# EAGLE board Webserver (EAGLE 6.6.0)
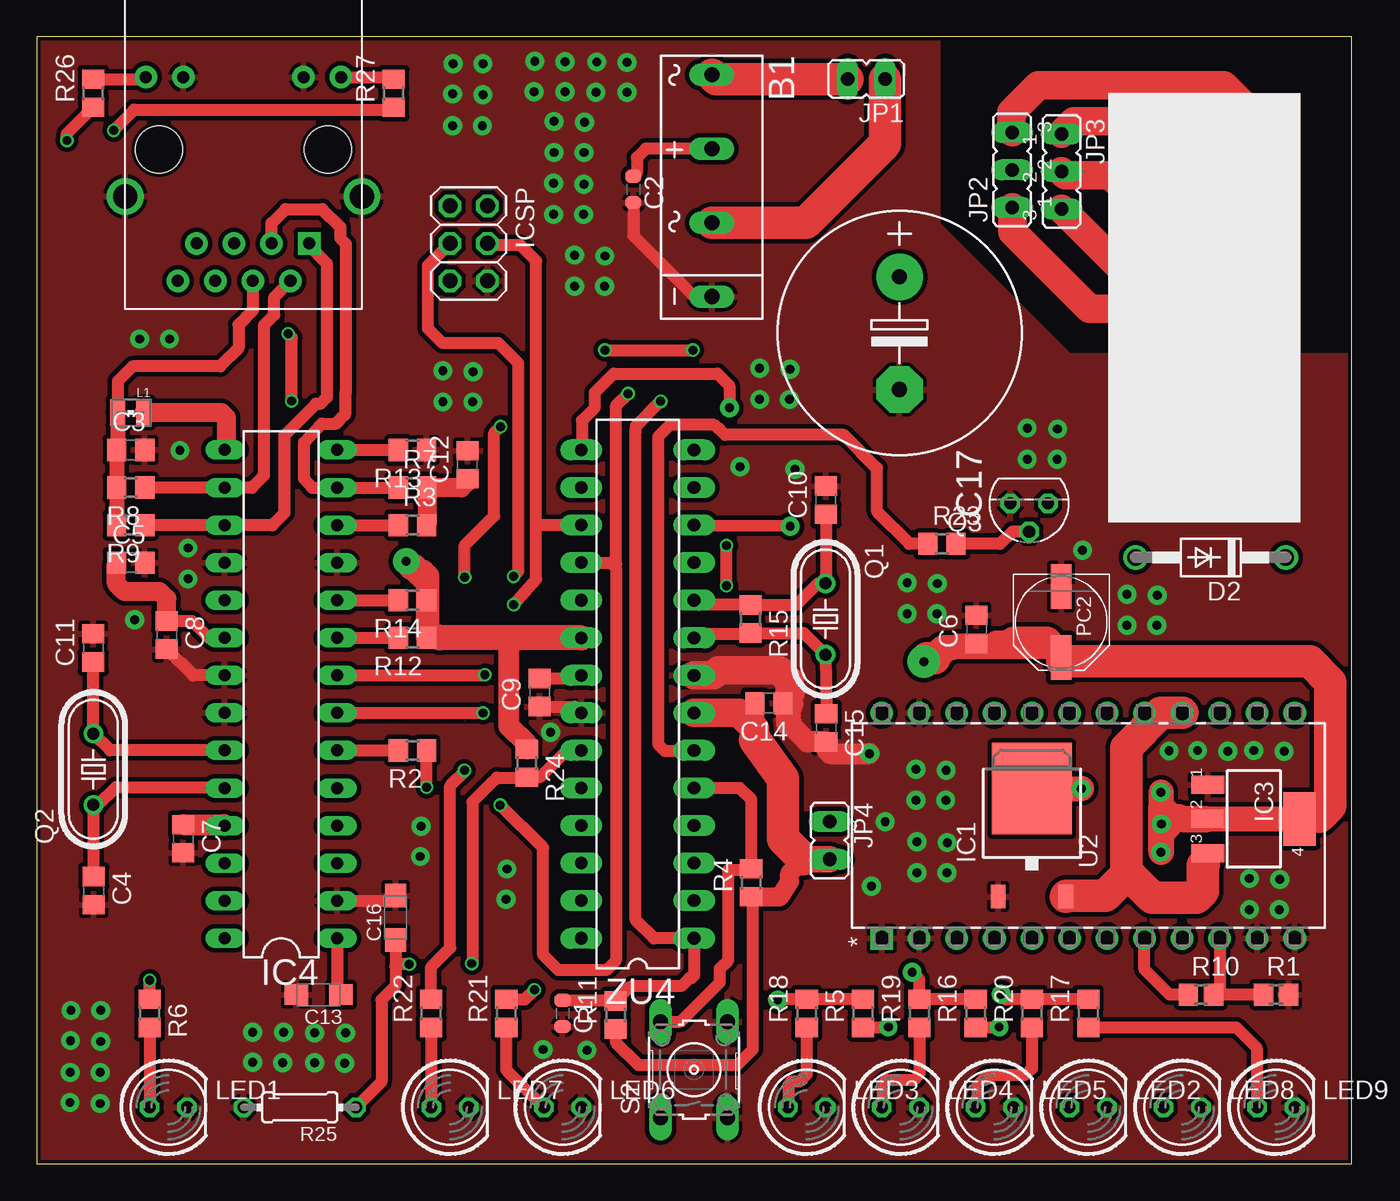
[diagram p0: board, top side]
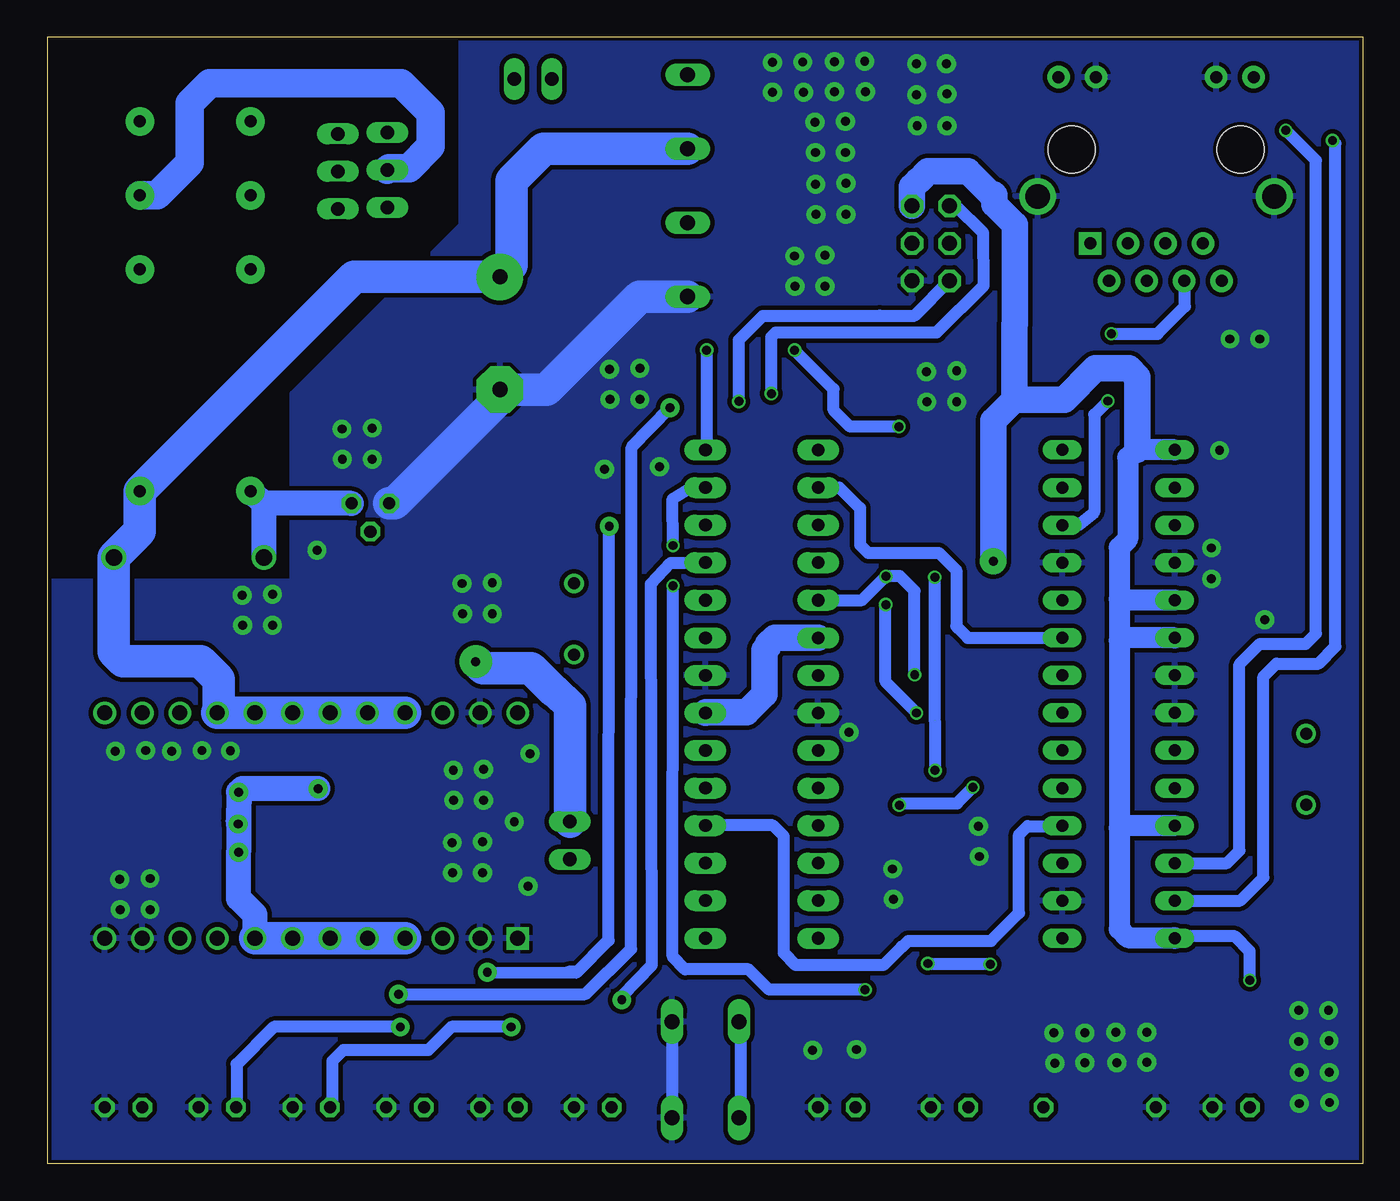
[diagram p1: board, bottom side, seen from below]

Size 88.95 x 76.19 mm. Coordinates in mm from the lower left corner, seen from the top.
Outline: 0,0 88.95,0 88.95,76.19 0,76.19 0,0
Copper layers (1*16): Top 0.035mm / dielectric 1.5mm / Bottom 0.035mm
Design rules "ITEADstudio_DRC *": minimum track width 6mil, minimum drill 12mil, track to track 12mil, track to pad 12mil, pad to pad 12mil, via to via 12mil, smd to smd 0mil, copper to edge 10mil, drill to drill 10mil, minimum pad ring 10mil, minimum via ring 6mil, stop-mask expansion 2mil, vias tented up to drill 100mil, thermal gap 10mil
Net classes: 0 default: width 0.152 mm, drill 0.305 mm, clearance 0.152 mm; 2 gnd: width 0.305 mm, drill 0.559 mm, clearance 0.254 mm; 3 usbvcc: width 0.508 mm, drill 0.61 mm, clearance 0.254 mm; 4 aref: width 0.406 mm, drill 0.61 mm, clearance 0.254 mm

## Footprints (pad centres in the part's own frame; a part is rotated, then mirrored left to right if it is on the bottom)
2KBB = drill 1.016 long: + -2.616,0; - 7.391,0; AC1 -7.62,0; AC2 2.413,0
C0603-ROUND = smd 0.898 x 1.1: 1 -0.889,0; 2 0.889,0
C0805 = smd 1.3 x 1.5: 1 -0.95,0; 2 0.95,0
SMC_A = smd 1.6 x 1.4: + -1.5,0; - 1.5,0
E7,5-16 = drill 1.016 pad 3.15: + -3.81,0 | drill 1.016 pad 3.15 octagon: - 3.81,0
DO41-10 = drill 1.118: A 5.08,0; C -5.08,0
DPACK = smd 1 x 1.6: 1 -2.28,-4.8; 3 2.28,-4.8 | smd 5.4 x 6.2: 2 0,2.5
SOT223 = smd 1.219 x 2.235: 1 -2.311,-3.099; 2 0,-3.099; 3 2.311,-3.099 | smd 3.6 x 2.2: 4 0,3.099
DIL28-3 = drill 0.813 long: 1 -16.51,-3.81; 2 -13.97,-3.81; 3 -11.43,-3.81; 4 -8.89,-3.81; 5 -6.35,-3.81; 6 -3.81,-3.81; 7 -1.27,-3.81; 8 1.27,-3.81; 9 3.81,-3.81; 10 6.35,-3.81; 11 8.89,-3.81; 12 11.43,-3.81; 13 13.97,-3.81; 14 16.51,-3.81; 15 16.51,3.81; 16 13.97,3.81; 17 11.43,3.81; 18 8.89,3.81; 19 6.35,3.81; 20 3.81,3.81; 21 1.27,3.81; 22 -1.27,3.81; 23 -3.81,3.81; 24 -6.35,3.81; 25 -8.89,3.81; 26 -11.43,3.81; 27 -13.97,3.81; 28 -16.51,3.81
2X03 = drill 1.016 octagon: 1 -2.54,-1.27; 2 -2.54,1.27; 3 0,-1.27; 4 0,1.27; 5 2.54,-1.27; 6 2.54,1.27
HR911105A = drill 0.813 pad 1.524 square: 1 4.445,-6.35 | drill 0.813 pad 1.524: 2 3.175,-8.89; 3 1.905,-6.35; 4 0.635,-8.89; 5 -0.635,-6.35; 6 -1.905,-8.89; 7 -3.175,-6.35; 8 -4.445,-8.89; 9 6.604,4.902; 10 4.064,4.902; 11 -4.064,4.902; 12 -6.604,4.902 | drill 1.651 pad 2.159: 13 8.001,-3.175; 14 -8.001,-3.175 | hole 3.2: 5.715,0; -5.715,0
JP1 = drill 0.914 long: 1 0,-1.27; 2 0,1.27
JP2 = drill 0.914 long: 1 -2.54,0; 2 0,0; 3 2.54,0
WE-KI_0805_B = smd 1.02 x 1.78: 1 -0.89,0; 2 0.89,0
LED5MM = drill 0.813 octagon: A -1.27,0; K 1.27,0
PANASONIC_D = smd 3 x 1.4: + 2.4,0; - -2.4,0
HC49/S = drill 0.813: 1 -2.413,0; 2 2.413,0
TO92 = drill 0.813 octagon: 1 1.27,0; 2 0,1.905; 3 -1.27,0
R2012 = smd 1.3 x 1.5: 1 -0.85,0; 2 0.85,0
R0805 = smd 1.3 x 1.5: 1 -0.95,0; 2 0.95,0
0204/7 = drill 0.813 octagon: 1 -3.81,0; 2 3.81,0
B3F-10XX = drill 1.016 long: 1 -3.251,2.261; 2 3.251,2.261; 3 -3.251,-2.261; 4 3.251,-2.261
NA24F = drill 1.016 square: 1 -15.24,27.94 | drill 1.016: 2 -15.24,25.4; 3 -15.24,22.86; 4 -15.24,20.32; 5 -15.24,17.78; 6 -15.24,15.24; 7 -15.24,12.7; 8 -15.24,10.16; 9 -15.24,7.62; 10 -15.24,5.08; 11 -15.24,2.54; 12 -15.24,0; 13 0,0; 14 0,2.54; 15 0,5.08; 16 0,7.62; 17 0,10.16; 18 0,12.7; 19 0,15.24; 20 0,17.78; 21 0,20.32; 22 0,22.86; 23 0,25.4; 24 0,27.94
AZ733_2C_12DA = drill 0.8 pad 1.93: CC1 22.1,2.75; CC2 22.1,10.25; L1 2.1,2.75; L2 2.1,10.25; OC1 27.1,2.75; OC2 27.1,10.25; SC1 17.1,2.75; SC2 17.1,10.25
DIL28-3' = drill 0.85 pad 1.422 long: 1 -16.51,-3.81; 2 -13.97,-3.81; 3 -11.43,-3.81; 4 -8.89,-3.81; 5 -6.35,-3.81; 6 -3.81,-3.81; 7 -1.27,-3.81; 8 1.27,-3.81; 9 3.81,-3.81; 10 6.35,-3.81; 11 8.89,-3.81; 12 11.43,-3.81; 13 13.97,-3.81; 14 16.51,-3.81; 15 16.51,3.81; 16 13.97,3.81; 17 11.43,3.81; 18 8.89,3.81; 19 6.35,3.81; 20 3.81,3.81; 21 1.27,3.81; 22 -1.27,3.81; 23 -3.81,3.81; 24 -6.35,3.81; 25 -8.89,3.81; 26 -11.43,3.81; 27 -13.97,3.81; 28 -16.51,3.81

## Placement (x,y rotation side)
B1  [2KBB]  45.66,66.03 270 top
C1  22p  [C0603-ROUND]  35.56,10.16 270 top
C2  100n  [C0603-ROUND]  40.35,65.88 270 top
C3  0.1uF  [C0805]  6.35,48.26 0 top
C4  27pf  [C0805]  3.84,18.46 270 top
C5  0.1uF  [C0805]  6.35,40.64 0 top
C6  0.1uF  [C0805]  63.56,36.13 90 top
C7  0.1uF  [C0805]  9.9,21.97 270 top
C8  0.1uF  [C0805]  8.78,35.75 270 top
C9  100n  [C0805]  34.01,31.86 90 top
C10  27pf  [C0805]  53.37,44.87 90 top
C11  27pf  [C0805]  3.81,34.88 90 top
C12  0.1uF  [C0805]  29.13,47.26 90 top
C13  10uF  [SMC_A]  19.05,11.43 180 top
C14  100n  [C0805]  49.52,31.14 180 top
C15  27pf  [C0805]  53.4,29.47 270 top
C16  10uF  [SMC_A]  24.26,16.63 90 top
C17  470uF  [E7,5-16]  58.35,56.16 270 top
D2  1N4004  [DO41-10]  79.4,40.99 180 top
IC1  MC33269D-5.0  [DPACK]  67.31,22.86 0 top
IC3  MC33269ST-5.0T3  [SOT223]  82.32,23.31 270 top
IC4  ENC28J60SP  [DIL28-3]  16.51,31.75 90 top
ICSP  ICSP  [2X03]  29.21,62.23 270 top
J3  HR911105A  [HR911105A]  13.97,68.58 0 top
JP1  [JP1]  56.1,73.34 90 top
JP2  [JP2]  65.97,67.2 90 top
JP3  [JP2]  69.31,67.1 270 top
JP4  [JP1]  53.62,21.85 180 top
L1  [WE-KI_0805_B]  6.35,50.8 180 top
LED1  [LED5MM]  8.89,3.81 0 top
LED2  [LED5MM]  71.12,3.81 0 top
LED3  [LED5MM]  52.07,3.81 0 top
LED4  [LED5MM]  58.42,3.81 0 top
LED5  [LED5MM]  64.77,3.81 0 top
LED6  [LED5MM]  35.56,3.81 0 top
LED7  [LED5MM]  27.94,3.81 0 top
LED8  [LED5MM]  77.47,3.81 0 top
LED9  [LED5MM]  83.82,3.81 0 top
PC2  47u  [PANASONIC_D]  69.29,36.62 270 top
Q1  16Mhz  [HC49/S]  53.34,36.83 270 top
Q2  25Mhz  [HC49/S]  3.81,26.67 90 top
Q3  BC547  [TO92]  67.12,44.65 180 top
R1  1K  [R2012]  83.82,11.43 0 top
R2  270  [R0805]  25.4,27.94 180 top
R3  49R9 1%  [R0805]  25.4,43.18 0 top
R4  10K  [R0805]  48.32,19 90 top
R5  410  [R0805]  55.88,10.16 90 top
R6  1K1  [R0805]  7.62,10.16 270 top
R7  49R9 1%  [R0805]  25.4,45.72 0 top
R8  49R9 1%  [R0805]  6.35,45.72 180 top
R9  49R9 1%  [R0805]  6.35,43.18 180 top
R10  1K  [R2012]  78.74,11.43 0 top
R11  10K  [R0805]  39.15,10.05 90 top
R12  10K  [R0805]  25.4,35.56 180 top
R13  2K32  [R0805]  25.4,48.26 180 top
R14  10K  [R0805]  25.4,38.1 180 top
R15  1M  [R0805]  48.26,36.83 270 top
R16  410  [R0805]  63.5,10.16 90 top
R17  410  [R0805]  71.12,10.16 90 top
R18  410  [R0805]  52.07,10.16 90 top
R19  410  [R0805]  59.69,10.16 90 top
R20  410  [R0805]  67.31,10.16 90 top
R21  510  [R0805]  31.75,10.16 90 top
R22  510  [R0805]  26.67,10.16 90 top
R23  5K  [R0805]  61.22,41.91 0 top
R24  2K  [R0805]  33.14,27.08 270 top
R25  2K  [0204/7]  17.78,3.81 180 top
R26  1K1  [R0805]  3.81,72.39 90 top
R27  1K1  [R0805]  24.13,72.39 90 top
S2  [B3F-10XX]  44.45,6.35 90 top
U2  LM2825N-ADJ  [NA24F]  85.09,30.48 90 top
U$1  AZ733_2C_12DA  [AZ733_2C_12DA]  85.47,43.38 90 top
ZU4  ATMEGA328P-PU  [DIL28-3']  40.64,31.75 90 top

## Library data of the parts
B1 = rectifier
C1 C2 ZU4 = SmartPrj
C3-C17 PC2 R1-R27 = rcl
D2 = diode
IC1 IC3 = linear
IC4 = microchip; MF: MICROCHIP; MPN: ENC28J60/SP; OC_FARNELL: 1084619; OC_NEWARK: 96K3661
ICSP = pinhead
J3 = CONNECTER
JP1-JP4 = jumper
L1 = wuerth-elektronik
LED1-LED9 = led
Q1 Q2 = crystal; OC_FARNELL: 1667008; OC_NEWARK: unknown
Q3 = transistor-npn
S2 = switch-omron; MPN: B3F-1000; OC_FARNELL: 176432; OC_NEWARK: 36M3542
U2 = LM2825N_ADJ; BASE_PN: LM2825; COMPTYPE: Switcher; MANUFACTURER_PART_NUMBER: LM2825N-ADJ; SYMBOL: NameLM2825N-ADJ; TYPE: LM2825N-ADJ; VENDOR: National; VERSION: 05/02/2007
U$1 = AZ733

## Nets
AD0: C16.+ R24.2 R25.1 ZU4.23
AREF [aref]: C9.2 ZU4.21
CCT: C3.1 J3.4 L1.2 R8.2 R9.2
ETH-CLK: IC4.8 ICSP.3 ZU4.19
ETH-CS: IC4.9 R12.2 ZU4.16
ETH-INT: IC4.4 ZU4.4
ETH-MISO: IC4.6 R2.2
ETH-MOSI: IC4.7 ICSP.4 ZU4.17
ETH-RST: IC4.10 R14.2
GND: B1.- C1.2 C2.2 C3.2 C4.2 C5.2 C6.2 C7.2 C8.2 C9.1 C10.2 C11.2 C12.2 C13.- C14.1 C15.2 C16.- C17.- IC1.1 IC3.1 IC4.2 IC4.11 IC4.18 IC4.21 IC4.22 ICSP.6 J3.10 J3.11 J3.13 J3.14 LED1.K LED2.K LED3.K LED4.K LED5.K LED6.K LED7.K LED8.K LED9.K PC2.- Q3.1 R1.2 R13.1 R25.2 S2.3 S2.4 U2.1 U2.2 U2.11 U2.12 U2.23 ZU4.8 ZU4.22
IO1: R5.2 R18.2 ZU4.11
IO2: R17.2 R20.2 ZU4.15
IO4: R23.1 ZU4.6
IO6: R16.2 R19.2 ZU4.12
IO7: R21.2 ZU4.13
IO8: R22.2 ZU4.14
LED_A: IC4.27 R26.1
LED_B: IC4.26 R27.1
LED_STATUS: J3.12 R26.2
MISO: ICSP.1 R2.1 ZU4.18
N$1: LED2.A R5.1
N$2: C4.1 IC4.24 Q2.1
N$3: C11.1 IC4.23 Q2.2
N$4: C12.1 R3.2 R7.2
N$5: IC4.14 R13.2
N$6: C15.1 Q1.2 R15.2 ZU4.9
N$7: LED1.A R6.2
N$8: C13.+ IC4.1
N$9: LED8.A R16.1
N$10: LED3.A R18.1
N$11: LED4.A R19.1
N$12: LED5.A R20.1
N$13: Q3.2 R23.2
N$14: JP3.3 U$1.SC2
N$15: LED6.A R21.1
N$16: LED7.A R22.1
N$17: D2.A Q3.3 U$1.L2
N$18: JP3.2 U$1.CC2
N$19: J3.9 R27.2
N$20: JP3.1 U$1.OC2
N$21: R1.1 R10.2 U2.10
N$22: B1.AC2 JP1.1
N$23: B1.AC1 JP1.2
N$24: JP2.2 U$1.CC1
N$25: JP2.1 U$1.SC1
N$26: JP2.3 U$1.OC1
N$27: R4.2 S2.1 S2.2 ZU4.5
N$29: LED9.A R17.1
N$30: IC1.2 IC3.2 IC3.4 R10.1 U2.4 U2.5 U2.6 U2.7 U2.8
RD+: IC4.13 J3.3 R7.1
RD-: IC4.12 J3.6 R3.1
RESET: C1.1 ICSP.5 R11.2 ZU4.1
S$1: C6.1
S$2: JP4.1
TD+: IC4.17 J3.1 R9.1
TD-: IC4.16 J3.2 R8.1
V+: C5.1 C7.1 C8.1 C14.2 IC4.15 IC4.19 IC4.20 IC4.25 IC4.28 ICSP.2 JP4.2 L1.1 R4.1 R6.1 R11.1 R12.1 R14.1 R24.1 ZU4.7 ZU4.20
VIN: B1.+ C2.1 C17.+ D2.C IC1.3 IC3.3 U2.16 U2.17 U2.18 U2.19 U2.20 U2.21 U$1.L1
XTAL2: C10.1 Q1.1 R15.1 ZU4.10

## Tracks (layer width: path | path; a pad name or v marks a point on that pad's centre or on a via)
AD0  (via drill 0.6)
  Top 0.813: C16.+ 24.26,13.33 | 24.26,13.33 24.26,12.02 23.31,11.07 23.31,5.53 R25.1 | 36.51,27.62 ZU4.23 36.81,27.96 35.85,27.96 34.02,26.13 R24.2 33.11,26.1 31.11,26.1 30.75,25.74 30.74,25.74 29.46,24.46 29.46,13.58 v29.41,13.53 | v25.18,13.48 24.41,13.48 24.26,13.33
  Bottom 0.813: v29.41,13.53 25.23,13.53 v25.18,13.48
AREF
  Top 0.813: C9.2 36.62,32.81 ZU4.21
CCT
  Top 0.813: J3.4 14.61,57.71 13.63,56.74 13.63,55.14 12.41,53.92 6.47,53.92 5.47,52.92 L1.2
  Top 1.016: L1.2 5.46,48.32 C3.1 R8.2 R9.2
ETH-CLK  (via drill 0.6)
  Top 0.813: IC4.8 30.26,33.02 v30.3,33.06 | 32.48,39.96 v32.24,39.72 v32.24,39.71 32.48,39.96 | 32.48,39.96 32.58,40.06 32.58,54.12 31.22,55.48 27.45,55.48 26.46,56.47 26.46,60.75 ICSP.3 27.86,62.15
  Bottom 0.813: ZU4.19 33.85,38.1 v32.24,39.71 32.22,39.73 31.3,39.73 30.3,38.73 v30.3,33.06
ETH-CS
  Top 0.813: IC4.9 R12.2
  Bottom 0.813: ZU4.16 35.39,45.72 33.99,44.32 33.99,41.85 33.45,41.31 28.66,41.31 27.48,40.13 27.48,36.37 27.38,36.27 27.38,36.23 26.7,35.55 IC4.9
ETH-INT
  Bottom 0.813: ZU4.4 39.89,22.87 39.15,22.13 39.15,14.25 38.33,13.43 32.42,13.43 31.17,14.68 31.11,14.68 30.73,15.06 25.13,15.06 23.24,16.95 23.24,22.25 22.66,22.83 20.35,22.83 IC4.4
ETH-MISO
  Top 0.813: IC4.6 R2.2
ETH-MOSI  (via drill 0.6)
  Top 0.813: 33.78,43 33.78,61.05 32.71,62.12 30.59,62.12 ICSP.4 | ZU4.17 33.96,43.18 33.78,43 | 33.78,43 33.78,39.53 v32.25,37.8 | IC4.7 v30.17,30.48 v30.18,30.47
  Bottom 0.813: v30.18,30.47 30.18,30.5 32.27,32.59 32.27,37.78 v32.25,37.8
ETH-RST
  Top 0.813: IC4.10 R14.2
GND  (via drill 0.6 pad 1.27)
  Top 0.61: 50.98,31.07 50.54,31.07 C14.1
  Top 0.813: IC4.2 23.61,17.78 C16.- | C2.2 40.35,62.76 44.42,58.69 45.61,58.69 B1.- | C9.1 36.4,30.91 ZU4.22 | IC4.21 10.56,33.02 C8.2 | 56.23,27.81 v56.31,27.73
  Top 1.27: 50.96,31.82 50.96,31.63 C14.1
  Top 1.422: C15.2 53.43,28.13 | v56.31,27.73 v56.3,27.73 53.67,27.73 53.42,27.98 53.42,28.49 C15.2 | C15.2 52.2,28.52 52.12,28.52 50.87,29.77
  Top 1.676: 50.87,29.77 50.87,29.87 50.84,29.9 50.84,30.7 50.86,30.72 50.86,30.95 50.98,31.07
  Top 1.93: ZU4.8 45.76,33.02 46.12,33.38 50.22,33.38 50.26,33.34 50.26,33.3 50.92,32.64 50.92,31.86 50.96,31.82
  Bottom 0.813: S2.4 S2.3
  Bottom 2.184: C17.- 57.79,52.35 | 57.79,52.35 55.19,52.35 48.91,58.63 B1.- | Q3.1 65.49,44.65 57.79,52.35
  other vias: 9.67,48.23 10.22,39.54 70.73,41.48 66.99,47.64 66.99,49.74 69.01,47.64 69.04,49.68 75.76,36.4 75.79,38.44 73.74,36.4 73.74,38.5 60.89,37.19 60.92,39.23 58.87,37.19 58.87,39.29 61.48,24.57 61.51,26.61 59.46,24.57 59.46,26.67 59.53,19.67 59.53,21.77 61.55,19.67 61.58,21.71 36.37,59.34 36.37,61.44 38.39,59.34 38.42,61.38 34.95,64.19 34.95,66.29 36.97,64.19 37,66.23 34.99,68.38 34.99,70.48 37.01,68.38 37.04,70.42 39.91,72.45 37.81,72.45 39.91,74.47 37.87,74.5 35.72,72.49 33.62,72.49 35.72,74.51 33.68,74.54 30.17,74.38 30.17,72.28 28.15,74.38 28.12,72.34 30.13,70.19 28.11,70.19 4.32,10.36 4.32,8.26 2.3,10.36 2.27,8.32 4.28,6.17 4.28,4.07 2.26,6.17 2.23,4.13 14.59,8.88 16.69,8.88 14.59,6.86 16.63,6.83 18.78,8.84 20.88,8.84 18.78,6.82 20.82,6.79 10.22,41.63 6.62,36.78 51.27,46.96 48.89,51.68 48.89,53.78 50.91,51.68 50.94,53.72 34.24,7.72 37.2,7.66 25.99,22.82 25.93,20.77 31.79,19.92 31.73,17.87 27.46,51.51 27.46,53.61 29.48,51.51 29.51,53.55 84.37,27.88 82.32,27.94 80.56,27.88 78.51,27.94 76.59,27.91 8.97,55.77 6.95,55.77 56.45,18.76 57.38,23.12 47.57,47.13 34.75,29.18 84.04,17.18 84.07,19.22 82.02,17.18 82.02,19.28
  pour Bottom: -1.27,77.47 -1.27,-1.27 90.17,-1.27 90.17,39.37 72.39,39.37 72.39,52.07 60.96,63.5 60.96,77.47
  pour Top: -1.27,78.74 -1.27,-1.27 90.17,-1.27 90.17,54.61 69.85,54.61 60.96,63.5 60.96,77.47 60.96,78.74
IO1  (via drill 0.6 pad 1.27)
  Top 0.813: R5.2 R18.2 49.85,11.11 v50.11,11.07
  Bottom 0.813: v50.11,11.07 50.11,11.31 48.08,13.42 48.14,39.2 46.8,40.62 44.47,40.62 ZU4.11
IO2  (via drill 0.6 pad 1.27)
  Top 0.813: R17.2 R20.2 65.57,11.11 v65.22,11.46 | ZU4.15 36.86,48.29 36.86,50.24 37.74,51.12 37.74,52.16 39.01,53.43 46.03,53.43 46.84,52.62 v46.84,51.13 v46.85,51.12
  Bottom 0.813: v65.22,11.46 52.59,11.46 49.47,14.52 49.44,48.44 v46.85,51.12
IO4
  Top 0.813: R23.1 59.02,41.91 56.84,44.09 56.84,47.04 54.59,49.29 46.55,49.29 46.14,49.7 46.09,49.7 45.83,49.96 42.84,49.96 42.02,49.14 42.02,28.37 42.47,27.92 44.43,27.92 ZU4.6
IO6  (via drill 0.6 pad 1.27)
  Top 0.813: R16.2 R19.2 59.69,12.46 v59.21,12.94 | v50.96,43.11 44.5,43.13 ZU4.12
  Bottom 0.813: v59.21,12.94 53.18,12.92 | 53.18,12.92 53.32,12.97 53.72,12.96 53.18,12.92 | 53.18,12.92 51,15.1 v50.96,43.11
IO7  (via drill 0.6)
  Top 0.813: R21.2 33,11.11 v33.65,11.76 | v46.65,39.08 v46.65,41.8
  Bottom 0.813: v33.65,11.76 40.15,11.76 41.53,13.14 45.82,13.14 46.67,14.01 v46.65,39.08 | v46.65,41.8 46.67,44.95 45.37,45.79 44.52,45.79 ZU4.13
IO8  (via drill 0.6)  (1 unrouted)
  Top 0.813: R22.2 26.67,13.3 27.96,14.59 27.96,25.54 28.98,26.56 v28.92,26.59 | v28.94,39.65 28.94,41.81 30.94,43.81 30.94,49.42 v31.36,49.84 | v38.42,55.01 v44.37,55.01
  Bottom 0.813: 28.94,29.96 v28.94,39.65 | v31.36,49.84 34.66,49.84 35.78,50.96 35.78,52.37 v38.42,55.01 | 28.93,29.95 v28.92,26.59 | v44.37,55.01 44.37,48.34 ZU4.14
LED_A  (via drill 0.6)
  Top 0.813: v2.03,69.19 2.03,69.66 R26.1
  Bottom 0.813: IC4.27 8.27,17.78 6.71,19.34 6.71,32.93 5.82,33.82 2.97,33.82 1.83,34.96 1.83,68.99 v2.03,69.19
LED_B  (via drill 0.6)
  Top 0.813: v5.19,69.87 5.19,69.89 6.57,71.27 23.96,71.27 R27.1
  Bottom 0.813: IC4.26 9.17,20.32 8.33,21.16 8.33,33.77 6.95,35.15 3.85,35.15 3.16,35.84 3.16,67.84 v5.19,69.87
LED_STATUS
  Top 0.813: R26.2 7.22,73.34 J3.12
MISO  (via drill 0.6)
  Top 0.813: v31.34,24.24 34.24,21.36 34.24,14.12 35.27,13.09 38.53,13.09 39.17,13.73 39.17,40.28 38.81,40.64 ZU4.18 39.11,40.64 39.19,40.56 39.19,51.27 v39.99,52.07 | v26.36,25.45 R2.1
  Bottom 0.813: v31.34,24.24 31.4,24.22 31.19,24.37 27.44,24.37 v26.36,25.45 | v39.99,52.07 39.99,55.91 39.69,56.21 28.82,56.21 25.63,59.4 25.65,62.92 27.56,64.8 ICSP.1
N$1  (via drill 0.6 pad 1.27)
  Top 0.813: R5.1 57.56,9.21 v57.59,9.24
  Bottom 0.813: v57.59,9.24 61.63,9.24 63.2,7.67 68.96,7.67 69.7,6.93 69.7,3.96 LED2.A
N$2
  Top 0.813: C4.1 3.84,24.23 Q2.1 4.13,24.26 5.33,25.46 12.64,25.46 IC4.24
N$3
  Top 0.813: IC4.23 4.95,27.94 Q2.2 C11.1
N$4
  Top 1.27: C12.1 29.13,46.12 28.7,45.69 26.38,45.69 | 26.38,45.69 R7.2 | 26.38,45.69 26.38,43.21 R3.2
N$5
  Top 0.813: IC4.14 R13.2
N$6
  Top 0.813: ZU4.9 44.53,35.56 44.79,35.82 48.2,35.82 R15.2 51.88,35.88 Q1.2 C15.1
N$7
  Top 0.813: R6.2 LED1.A
N$8
  Top 0.813: IC4.1 20.32,11.66 C13.+
N$9  (via drill 0.6 pad 1.27)
  Top 0.813: R16.1 65.06,9.21 v65.09,9.24
  Bottom 0.813: v65.09,9.24 73.66,9.24 76.17,6.73 76.17,3.84 LED8.A
N$10
  Top 0.813: R18.1 52.07,6.04 51.58,5.55 51.04,5.55 50.84,5.35 50.84,3.85 LED3.A
N$11
  Top 0.813: R19.1 59.69,6.03 59.31,5.65 57.44,5.65 57.19,5.4 57.19,3.85 LED4.A
N$12
  Top 0.813: R20.1 67.31,6.44 66.86,5.99 64.3,5.99 63.61,5.3 63.61,3.92 LED5.A
N$13
  Top 0.813: Q3.2 66.01,42.74 65.17,41.91 R23.2
N$14
  Top 1.93: U$1.SC2 73.39,60.48 JP3.3
N$15
  Top 0.813: R21.1 31.75,6.35 LED6.A
N$16
  Top 0.813: R22.1 LED7.A
N$17
  Bottom 1.676: D2.A 74.32,44.58 | 74.32,44.58 U$1.L2 | Q3.3 74.25,44.65 74.32,44.58
N$18
  Top 1.93: U$1.CC2 73.98,65.48 72.61,66.85 69.56,66.85 JP3.2
N$19
  Top 0.813: J3.9 23.99,73.48 R27.2
N$20
  Top 1.93: U$1.OC2 70.15,70.48 JP3.1
N$21
  Top 0.813: U2.10 80.01,11.85 79.94,11.78 | 79.94,11.78 R10.2 | R1.1 80.29,11.43 79.94,11.78
N$22
  Top 2.184: B1.AC2 52.01,63.62 57.37,68.98 JP1.1
N$23
  Top 2.184: JP1.2 45.97,73.34 B1.AC1
N$24
  Bottom 1.93: U$1.CC1 81.55,65.48 79.35,67.68 79.35,71.7 77.99,73.06 65.04,73.06 63.03,71.05 63.03,68.8 64.51,67.32 65.85,67.32 JP2.2
N$25
  Top 1.93: JP2.1 65.97,63.02 71.19,57.8 80.04,57.8 U$1.SC1
N$26
  Top 1.93: U$1.OC1 82.72,70.51 80.29,72.94 67.76,72.94 65.93,71.11 65.93,69.78 JP2.3
N$27
  Top 0.813: ZU4.5 47.54,25.4 48.32,24.62 R4.2 48.24,19.87 46.77,19.87 46.77,13.77 46.2,13.2 46.2,12.26 43.54,9.6 S2.2
  Bottom 0.813: S2.2 42.19,9.28 42.09,9.18 42.09,3.2 S2.1
N$28
  Bottom 1.676: 76.01,24.79 76.06,23.03 76.02,23.3 76.01,24.79
N$29
  Top 0.813: R17.1 81.13,9.21 82.52,7.82 82.52,3.84 LED9.A
N$30  (via drill 0.6 pad 1.27)
  Top 0.813: R10.1 76.63,11.43 74.92,13.14 U2.8
  Top 1.676: IC3.2 76.68,23.31 76.65,23.34 76.65,22.89 76.07,22.31 76.07,21.09 v76.03,21.05 76.03,24.2 | 76.03,24.2 76.75,23.48 77.26,23.48 77.47,23.27 79.2,23.27 79.24,23.31 IC3.4 | IC1.2 v70.66,25.36 | v76.03,25.12 76.03,24.2
  Bottom 1.676: U2.8 74.93,16.84 76.03,17.94 v76.03,21.05 76.03,23.16 v76.06,22.97 | v70.66,25.36 75.79,25.36 v76.03,25.12
  Bottom 2.184: U2.4 U2.5 U2.6 U2.7 U2.8
RD+
  Top 0.813: J3.3 15.88,63.61 16.82,64.55 19.3,64.55 20.51,63.34 20.51,62.58 20.89,62.2 20.89,52.14 20.88,52.13 20.88,50.72 20.82,50.66 20.82,50.63 20.24,50.05 19.26,50.05 18.06,48.77 18.06,46.33 18.63,45.7 20.3,45.7 IC4.13 R7.1
RD-  (via drill 0.6)
  Top 0.813: IC4.12 R3.1 | v17.23,51.57 17.23,55.88 v16.99,56.12
  Bottom 0.813: IC4.12 19.2,43.19 18.15,44.06 18.15,50.65 v17.23,51.57 | v16.99,56.12 13.87,56.12 12.02,57.97 12.02,59.64 J3.6
RESET  (via drill 0.6)
  Top 0.813: C1.1 35.61,11 R11.2 40.05,11.9 40.2,11.9 40.3,12 43.59,12 44.13,12.54 44.28,12.54 44.45,12.71 ZU4.1 41.73,15.24 40.5,16.47 40.5,49.48 40.51,49.87 v42.19,51.55
  Bottom 0.813: ICSP.5 30.29,57.34 32.65,57.34 32.66,57.33 40.56,57.33 42.19,55.7 v42.19,51.55
S$1  (via drill 0.6 pad 2.18)
  Top 0.406: 69.37,33.97 68.13,35.21 68.07,35.21 68.04,35.18 C6.1
  Top 1.27: 64.92,35.21 64.89,35.18 C6.1 62.24,35.18 61.95,34.89
  Top 1.676: 66.12,35.24 66.09,35.21 64.92,35.21 | 61.95,34.89 61.45,34.89 61.3,34.74
  Top 1.93: 61.3,34.74 61.27,34.74 60.7,34.17
  Top 2.184: 86.76,23.46 87.49,24.19 87.49,32.57 86.09,33.97 69.37,33.97 | 66.12,35.24 68.27,35.24 | 60.7,34.17 60.21,34.17 v59.99,33.95
S$2
  Bottom 2.184: 59.98,33.98 59.5,33.5 56.24,33.5 54.7,31.96 54.61,31.96 53.62,30.97 JP4.1
TD+
  Top 0.813: R9.1 IC4.17 15.92,43.17 16.75,44 16.75,49.27 18.88,51.4 19.2,51.4 19.61,51.81 19.61,60.87 18.41,62.06 J3.1
TD-
  Top 0.813: R8.1 IC4.16 12.72,45.7 14.53,45.7 15.35,46.52 15.35,56.69 16.06,57.4 16.06,58.6 J3.2
V+  (via drill 0.6, 0.6 pad 1.78)
  Top 0.813: 12.57,15.11 IC4.28 | IC4.20 11.62,35.56 10.49,36.69 C8.1 | R11.1 39.15,8.22 40.69,6.68 47.39,6.68 48.43,7.72 48.43,17.94 R4.1 | R6.1 v7.62,12.39 v7.63,12.4
  Top 1.27: L1.1 12.47,50.8 12.81,50.46 12.81,48.37 IC4.15 | 48.58,28.67 48.58,29.4 C14.2 | R4.1 48.34,18.03 50.22,18.03 50.92,19.09 50.92,19.62 51.87,20.58 | 27.18,35.62 26.41,35.62 R12.1 | C8.1 8.78,38.2 8.3,38.68 5.91,38.68 5.37,39.22 5.37,40.61 C5.1
  Top 1.422: C7.1 12.64,22.92 IC4.25 | R12.1 R14.1 26.35,39.38 26.34,39.39 26.34,39.47 25.85,39.96 | R24.1 33.14,28.38 31.93,29.59 31.93,35.11 31.48,35.56
  Top 1.676: ZU4.20 31.48,35.56 27.24,35.56 27.18,35.62
  Top 1.778: 25.85,39.96 26.04,39.96 26.32,39.68 26.17,39.68 25.51,40.34 25.37,40.34 v24.98,40.73 | 51.87,20.58 JP4.2
  Top 1.93: ZU4.7 47.5,30.48 48.58,29.4
  Top 2.184: 48.58,28.67 50.45,26.04 50.47,25.09 50.47,21.97 51.87,20.58
  Bottom 0.813: v7.63,12.4 7.63,14.37 8.62,15.36 12.58,15.36 IC4.28
  Bottom 1.422: IC4.15 15.28,48.26 15.38,48.26 15.89,47.75 15.89,42.23 16.46,41.66 16.46,38.18 | 16.46,38.18 16.46,35.39 | 16.46,35.39 16.46,22.68 | 16.46,22.68 16.46,15.88 15.87,15.29 12.75,15.29 IC4.28 | IC4.25 16.28,22.86 16.46,22.68 | IC4.19 16.38,38.1 16.46,38.18 | IC4.20 16.29,35.56 16.46,35.39
  Bottom 1.778: v24.98,40.73 24.98,50.24 23.56,51.66 | 23.56,51.66 20.18,51.66 18.06,53.78 15.81,53.78 15.22,53.19 15.22,48.32 15.28,48.26 | 23.56,51.66 23.56,56.73 23.51,56.78 23.51,63.49 24.9,64.88 24.9,65.48 24.96,65.54 25.14,65.54 26.7,67.1 29.39,67.1 30.02,66.47 30.08,66.47 30.5,66.05 30.5,64.79 ICSP.2 | ZU4.20 39.76,35.56 40.21,35.11 40.21,34.97 40.47,34.71 40.47,31.73 41.67,30.53 44.4,30.53 ZU4.7
VIN
  Top 0.813: B1.+ 41.2,68.65 40.58,68.03 40.58,67 C2.1
  Top 1.016: 78.94,20.25 78.94,20.72 IC3.3
  Top 2.184: U2.16 76.04,30.48 73.69,28.13 73.69,19.54 | 73.69,19.54 72.27,18.12 69.65,18.12 IC1.3 | 73.69,19.54 73.9,19.54 75.46,17.98 78.44,17.98 78.87,18.41 78.87,20.18 78.94,20.25
  Bottom 2.184: B1.+ 55.39,68.65 57.57,66.47 57.57,60.75 C17.+ 68.23,59.97 U$1.L1 82.72,42.75 D2.C 84.48,34.6 83.84,33.96 78.59,33.96 77.38,32.75 77.38,30.57 U2.16 U2.17 U2.18 U2.19 U2.20 U2.21
XTAL2
  Top 0.813: C10.1 53.37,39.27 Q1.1 52.83,39.24 51.36,37.77 R15.1 44.77,37.78 ZU4.10
(copper drawn outside any net)
  shapes: Top area x2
